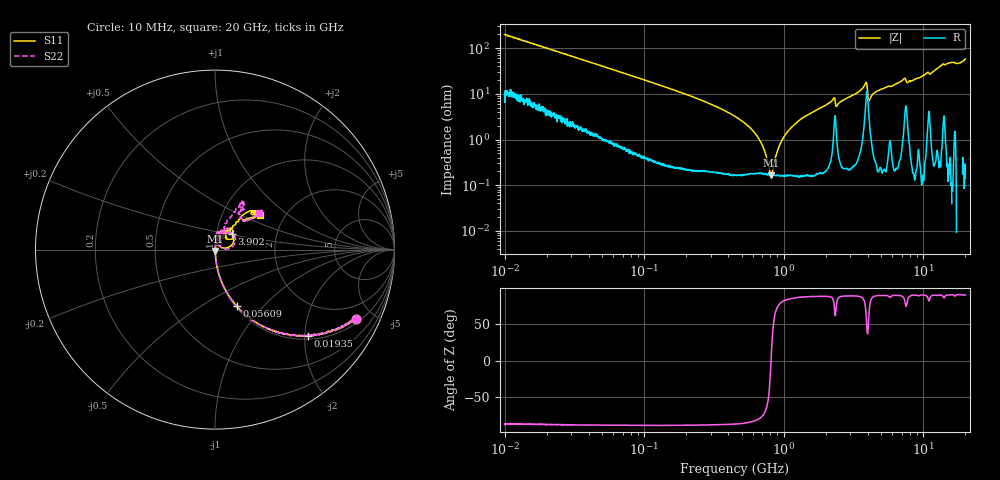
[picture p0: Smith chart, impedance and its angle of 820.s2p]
!Keysight Technologies,P5008B,MY61100088,A.16.20.02
!Date: Friday, August 30, 2024 14:33:08
!Correction: S11(C  2-Port  )
!S21(C  2-Port  )
!S12(C  2-Port  )
!S22(C  2-Port  )
!S2P File: Measurements: S11, S21, S12, S22:Log Frequency Sweep
# Hz S  MA  R 50
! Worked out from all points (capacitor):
!   1601 points, 10 MHz to 20 GHz, reference 50 ohm
!   read as one part in series: C = 80.2 pF near 10.39 MHz
!   lowest |Z| = 166 mohm at 809.9 MHz (marker M1)
!   series resonance near 810.2 MHz, so ESL is about 480 pH
!   S11 on the Smith chart (normalised r, x): 10 MHz: 1.18, -3.97; 19.35 MHz: 1.08, -2.06; 56.09 MHz: 1.02, -0.72; 3.902 GHz: 1.19, +0.21; 20 GHz: 1.51, +0.65
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1e7  0.8773 -26.2  0.4414 61.1  0.4415 61.1  0.8768 -26.2
1.935428e7  0.7043 -43.0  0.682 44.7  0.6819 44.7  0.704 -43.0
3.555162e7  0.4868 -59.1  0.8588 29.1  0.8586 29.1  0.4868 -59.2
5.609462e7  0.3368 -69.0  0.9336 19.6  0.9335 19.6  0.3367 -69.0
1.263918e8  0.1575 -79.9  0.9846 8.9  0.9843 8.9  0.1575 -80.2
4.472136e8  0.03656 -84.9  0.9977 1.6  0.9974 1.6  0.03644 -87.2
8.098563e8  0.008306 -72.7  0.9983 -0.4  0.998 -0.5  0.00784 -87.0
8.821543e8  0.005023 -60.1  0.9982 -0.7  0.9981 -0.7  0.004265 -86.8
9.654822e8  0.00234 -0.0  0.9983 -1.0  0.9982 -1.1  0.0005503 6.0
1.046689e9  0.004956 54.6  0.9983 -1.3  0.9981 -1.4  0.004046 85.0
1.129349e9  0.008476 62.9  0.9984 -1.6  0.9981 -1.6  0.007656 92.3
1.589917e9  0.02403 81.3  0.9982 -3.1  0.9979 -3.1  0.02373 85.4
2.238313e9  0.05116 76.4  0.9925 -5.4  0.9923 -5.5  0.05005 78.2
2.449743e9  0.03511 79.4  0.9948 -4.8  0.9945 -4.9  0.03476 73.8
3.902191e9  0.1291 42.3  0.9107 -10.5  0.9103 -10.6  0.1331 35.5
4.190402e9  0.03667 71.6  0.9879 -7.3  0.9876 -7.4  0.03909 55.4
5.652411e9  0.07401 73.1  0.993 -12.6  0.9929 -12.7  0.07641 71.4
7.27077e9  0.1253 52.7  0.9773 -17.5  0.9769 -17.6  0.1141 72.9
8.344716e9  0.0788 56.9  0.9977 -18.1  0.9977 -18.3  0.07636 80.9
9.441767e9  0.08958 55.4  0.9971 -21.2  0.9966 -21.4  0.08551 75.4
1.400536e10  0.2967 42.8  0.9393 -33.5  0.9391 -33.7  0.2745 55.8
2e10  0.3175 37.3  0.9505 -51.3  0.9506 -51.7  0.3203 39.4
